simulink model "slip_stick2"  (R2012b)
settings: Solver=ode1  StartTime=0.0  StopTime=100  FixedStep=0.001  MaxStep=0.001  RelTol=1e-3
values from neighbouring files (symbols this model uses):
  c = 2200    [coulomb_1.m]    (also in coulomb_10.m = 0.1; coulomb_11.m = 0; coulomb_2.m; coulomb_3.m)
  k = 10    [coulomb_10.m]    (also in coulomb_11.m; diff_filter_1.m = 250; diff_filter_2.m = 250; dry_friction_1.m = 2200)
  m = 400    [coulomb_1.m]    (also in coulomb_10.m = 10; coulomb_11.m = 10; coulomb_2.m; coulomb_3.m)
  vz = -ampl*2*pi*fanr*sin(2*pi*fanr*t)    [foerder_haft_gleit_1.m]    (also in foerder_haft_gleit_2.m; slip_stick_1.m = 0.1; slip_stick_2.m = 0.1; slip_stick_21.m = 0.1)

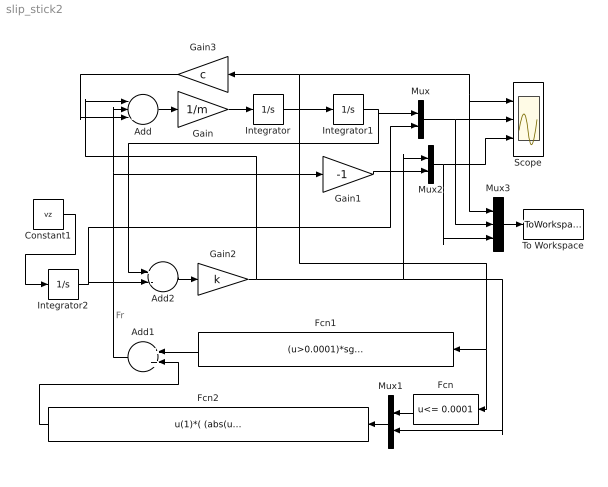
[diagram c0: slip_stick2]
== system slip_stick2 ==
  note: Fr
  Add : Sum  Inputs=---
  Add1 : Sum
  Add2 : Sum  Inputs=+-
  Constant1 : Constant  Value=vz
  Fcn : Fcn  Expr=u<= 0.0001
  Fcn1 : Fcn  Expr=(u>0.0001)*sgn(u)*(FG+(FH-FG)*exp(-abs(u/vstr)))
  Fcn2 : Fcn  Expr=u(1)*( (abs(u(2))>FH)*(-FH*sgn(u(2))) + (abs(u(2))<=FH)*(-u(2)) )
  Gain : Gain  Gain=1/m
  Gain1 : Gain  Gain=-1
  Gain2 : Gain  Gain=k
  Gain3 : Gain  Gain=c
  Integrator : Integrator
  Integrator1 : Integrator
  Integrator2 : Integrator
  Mux : Mux  Inputs=2
  Mux1 : Mux  Inputs=2
  Mux2 : Mux  Inputs=2
  Mux3 : Mux  Inputs=3
  Scope : Scope  NumInputPorts=3
  To Workspace : ToWorkspace  VariableName=y  SampleTime=-1  SaveFormat=Structure With Time
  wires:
  Add/1 -> Gain/1
  Gain/1 -> Integrator/1
  Gain3/1 -> Add/3
  Constant1/1 -> Integrator2/1
  Integrator2/1 -> Mux/2, Add2/2
  Add2/1 -> Gain2/1
  Integrator1/1 -> Mux/1, Add2/1
  Mux/1 -> Scope/2, Mux3/2
  Fcn1/1 -> Add1/1
  Fcn/1 -> Mux1/1
  Mux1/1 -> Fcn2/1
  Fcn2/1 -> Add1/2
  Mux2/1 -> Mux3/3, Scope/3
  Add1/1 -> Gain1/1, Add/2
  Gain2/1 -> Mux2/1, Mux1/2, Add/1
  Mux3/1 -> To Workspace/1
  Integrator/1 -> Fcn/1, Fcn1/1, Integrator1/1, Mux3/1, Scope/1, Gain3/1
  Gain1/1 -> Mux2/2
